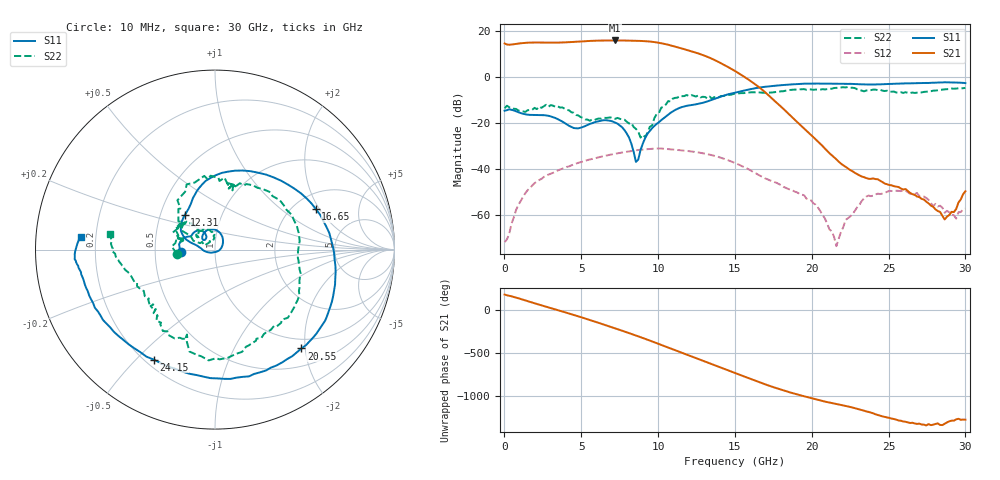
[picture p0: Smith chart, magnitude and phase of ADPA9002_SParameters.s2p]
! Analog Devices, Inc.
! Device:	ADPA9002
! Description:	GaAs PHEMT MMIC 2 Watt POWER AMPLIFIER, DC - 10 GHz
! Conditions:	Vdd = 12.0 V
!		Vgg1= GND
!		Idd = 385 mA quiescent (Self-biased mode)
!		Pin = -15 dBm
!		Operating Temperature = +25 C (at package bottom)
! Product validation unit SN11 soldered down to Evaluation Board as shown on ADPA9002-EVALZ User Guide. Board loss de-embedded from S21 magnitude.  All other RF measurements reference to RF coaxial connector.
! Frequency (GHz)	S11_Mag (dB)	S11_Phase (deg)	S21_Mag (dB)	S21_Phase (deg)	S12_Mag (dB)	S12_Phase (deg)	S22_Mag (dB)	S22_Phase (deg)
#  GHZ  S  DB  R 50
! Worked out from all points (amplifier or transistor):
!   201 points, 10 MHz to 30 GHz, reference 50 ohm
!   highest |S21| = 16.1 dB at 7.208 GHz (marker M1)
!   |S21| within 3 dB of that: start of sweep to 11.28 GHz
!   unconditionally stable (mu >= 1): start of sweep to end of sweep
!   at 4.958 GHz: K = 5.67, MAG = 15.8 dB, |S12| = -36.9 dB
!   at 15 GHz: K = 16.57, MAG = 4.8 dB, |S12| = -37.3 dB
!   at 30 GHz: K = 30551.15, MAG = -44.1 dB, |S12| = -57.2 dB
!   S11 on the Smith chart (normalised r, x): 10 MHz: 0.68, -0.02; 12.31 GHz: 0.67, +0.27; 16.65 GHz: 2.60, +1.86; 20.55 GHz: 0.81, -1.93; 24.15 GHz: 0.23, -0.56; 30 GHz: 0.14, +0.05
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0.01  -14.48 -176.6  14.77 178.3  -71.70 168.9  -13.44 -173.9
0.9097  -15.15 156.2  14.74 134.8  -55.47 117.7  -14.43 160.4
1.95935  -16.35 148.5  15.20 76.8  -46.04 46.8  -13.24 162.5
2.85905  -16.70 134.3  15.15 27.8  -42.33 -4.1  -12.79 144.1
3.6088  -18.63 122.7  15.18 -10.5  -40.16 -40.7  -13.12 140.3
5.1083  -21.57 140.0  15.72 -92.5  -36.60 -116.4  -17.66 135.4
6.3079  -18.79 116.5  16.06 -162.0  -34.45 -179.3  -17.97 143.5
7.2076  -19.68 80.8  16.10 144.5  -33.26 133.1  -18.05 124.7
7.8074  -22.91 51.8  16.07 107.8  -32.53 101.3  -18.39 108.5
8.4072  -32.36 -10.8  15.97 70.6  -31.91 68.7  -21.59 92.0
9.3069  -24.58 -172.1  15.72 12.4  -31.24 18.5  -24.11 158.7
10.05665  -19.48 166.9  15.07 -38.4  -30.94 -25.4  -15.42 150.6
10.95635  -14.78 158.9  13.69 -99.8  -31.39 -78.1  -9.23 127.3
12.3059  -11.86 131.3  11.11 170.3  -32.34 -154.1  -7.96 87.2
13.35555  -10.09 113.0  8.56 98.0  -33.63 146.0  -8.35 74.2
15.15495  -6.39 65.7  2.18 -26.3  -37.64 43.6  -7.18 43.0
16.65445  -4.36 22.0  -4.71 -126.8  -42.88 -42.0  -6.60 2.9
20.1033  -2.68 -41.8  -26.00 44.8  -54.80 121.0  -5.39 -52.2
20.55315  -2.71 -48.8  -28.91 24.5  -58.11 95.0  -5.29 -60.0
24.15195  -3.08 -119.1  -44.27 -137.2  -50.94 -176.0  -5.32 -118.8
25.05165  -2.84 -138.0  -46.85 -179.1  -49.39 156.1  -6.25 -131.4
30  -2.47 174.5  -49.56 160.9  -57.16 138.2  -4.56 171.4
